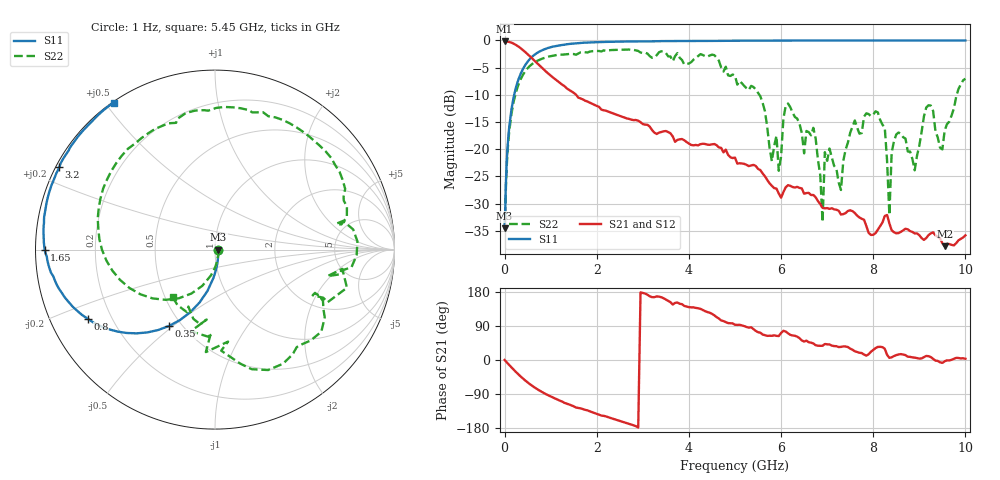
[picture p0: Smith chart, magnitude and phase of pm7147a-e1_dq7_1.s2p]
# GHz S DB R 50
! S-Parameters data
! Freq  dbS11  angS11  dbS21  angS21  dbS12  angS12  dbS22  angS22
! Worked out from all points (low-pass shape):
!   279 points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, 1 Hz to 10 GHz, reference 50 ohm
!   highest |S21| = -0.16 dB at 199.5 Hz (marker M1); lowest = -37.8 dB at 9.55 GHz (marker M2)
!   |S21| within 3 dB of the highest: start of sweep to 579.3 MHz
!   lowest |S11| = -34.6 dB at 158.5 Hz (marker M3), VSWR 1.04, Z = 51.9 - j2.19e-05 ohm
!   |S11| at or under -10 dB: start of sweep to 207.5 MHz
!   |S22| runs from -34.6 to -1.7 dB; largest |S21 - S12| = 0
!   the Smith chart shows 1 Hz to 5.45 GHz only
!   S11 on the Smith chart (normalised r, x): 1 Hz: 1.04, -0.00; 350 MHz: 0.43, -0.48; 800 MHz: 0.11, -0.25; 1.65 GHz: 0.03, +0.00; 3.2 GHz: 0.01, +0.25; 5.45 GHz: 0.00, +0.52
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1e-09  -34.57 -0.0  -0.16 -0.0  -0.16 -0.0  -34.57 -0.0
1.585e-07  -34.57 -0.0  -0.16 -0.0  -0.16 -0.0  -34.57 -0.0
1.995e-07  -34.57 -0.0  -0.16 -0.0  -0.16 -0.0  -34.57 -0.0
0.1  -15.97 -93.3  -0.28 -13.2  -0.28 -13.2  -16.75 -98.9
0.35  -6.09 -121.0  -1.44 -43.7  -1.44 -43.7  -7.10 -142.0
0.8  -1.86 -151.4  -4.95 -83.7  -4.95 -83.7  -3.40 165.0
1.65  -0.46 180.0  -10.67 -127.6  -10.67 -127.6  -2.18 102.1
1.7  -0.43 178.7  -10.85 -129.6  -10.85 -129.6  -2.13 98.2
3.2  -0.16 152.1  -16.47 165.9  -16.47 165.9  -3.20 11.9
3.35  -0.13 149.9  -16.95 167.3  -16.95 167.3  -2.18 8.3
5.05  -0.05 129.0  -22.65 92.6  -22.65 92.6  -8.12 -96.8
5.45  -0.06 124.6  -23.07 76.8  -23.07 76.8  -9.01 -131.7
5.95  -0.02 119.7  -28.14 63.2  -28.14 63.2  -23.97 -158.0
6.1  -0.02 118.2  -27.02 75.2  -27.02 75.2  -12.06 -100.1
6.7  -0.01 112.6  -28.41 43.6  -28.41 43.6  -16.06 170.8
6.9  -0.01 110.8  -30.79 37.5  -30.79 37.5  -33.39 -30.7
6.95  -0.01 110.4  -30.86 42.3  -30.86 42.3  -20.54 -138.1
8.1  -0.00 101.0  -34.80 34.5  -34.80 34.5  -13.23 -138.8
8.35  -0.01 99.1  -33.62 5.7  -33.62 5.7  -32.09 -87.3
8.5  -0.00 98.1  -35.47 12.9  -35.47 12.9  -17.29 -154.8
9.55  -0.00 90.9  -37.83 -3.4  -37.83 -3.4  -16.57 164.7
10  -0.00 88.1  -35.84 3.2  -35.84 3.2  -7.03 119.8
